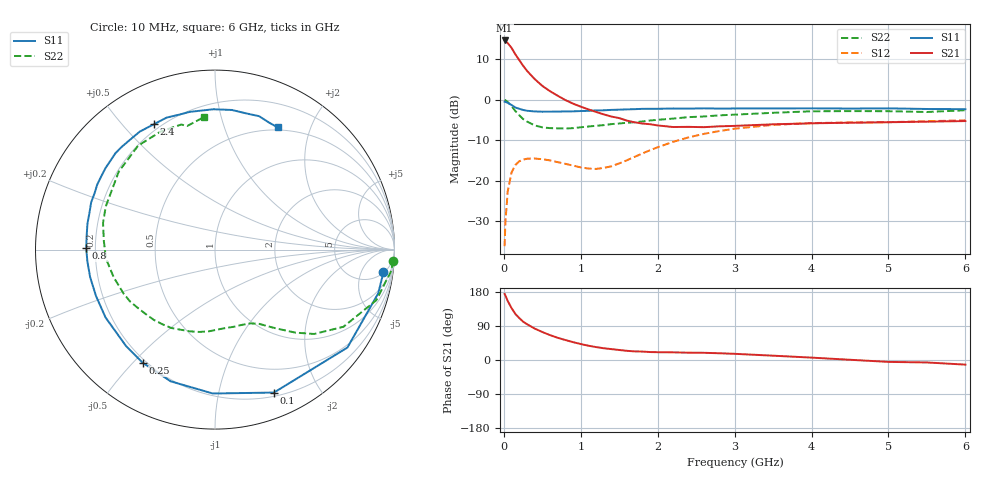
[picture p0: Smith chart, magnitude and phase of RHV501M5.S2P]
! SIEMENS Small Signal Semiconductors
! BFR106
! Si NPN RF Bipolar Junction Transistor in SOT23
! VCE = 0.5 V  IC = 1.5 mA
! Common Emitter S-Parameters:  August  1996
# GHz  S  MA  R  50
!  f  S11  S21  S12  S22
! GHz  MAG  ANG  MAG  ANG  MAG  ANG  MAG  ANG
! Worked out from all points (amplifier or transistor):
!   36 points, 10 MHz to 6 GHz, reference 50 ohm
!   highest |S21| = 14.7 dB at 10 MHz (marker M1)
!   |S21| within 3 dB of that: start of sweep to 136.2 MHz
!   unconditionally stable (mu >= 1): 770.4 MHz to end of sweep
!   at 250 MHz: K = 0.33, MSG = 11.6 dB, |S12| = -14.8 dB
!   at 1.4 GHz: K = 1.50, MAG = 2.0 dB, |S12| = -16.5 dB
!   at 6 GHz: K = 1.03, MAG = -1.1 dB, |S12| = -5.1 dB
!   S11 on the Smith chart (normalised r, x): 10 MHz: 5, -13; 100 MHz: 0.24, -1.47; 250 MHz: 0.19, -0.53; 800 MHz: 0.16, +0.01; 2.4 GHz: 0.17, +0.61; 6 GHz: 0.47, +1.53
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0.01  0.947 -7.6  5.425 174.4  0.0154 86.7  0.9962 -3.6
0.02  0.9415 -15.0  5.36 170.4  0.0302 83.4  0.9866 -7.3
0.05  0.9176 -36.5  5.041 155.9  0.0728 68.7  0.9421 -17.4
0.1  0.8616 -67.6  4.394 137.1  0.1258 52.4  0.835 -31.0
0.15  0.8018 -90.9  3.649 121.4  0.1559 39.7  0.7253 -40.4
0.2  0.7743 -108.6  3.104 110.8  0.173 31.6  0.6443 -45.9
0.25  0.7482 -122.6  2.646 101.3  0.1816 25.2  0.5779 -50.4
0.3  0.731 -132.7  2.288 94.6  0.1863 21.1  0.5379 -53.7
0.4  0.7176 -148.2  1.808 83.0  0.1873 14.8  0.4818 -59.2
0.5  0.7117 -158.6  1.487 73.9  0.1839 10.8  0.4559 -64.4
0.6  0.7124 -167.6  1.278 65.7  0.1776 8.7  0.4457 -70.0
0.8  0.7175 179.4  0.992 52.7  0.1611 8.7  0.4408 -82.2
1.1  0.7293 163.4  0.76 37.7  0.1408 18.8  0.4669 -100.7
1.6  0.7608 143.2  0.552 24.2  0.1782 44.9  0.5195 -131.2
2.2  0.7797 122.5  0.46 20.2  0.3015 46.8  0.585 -164.7
2.4  0.7771 115.8  0.462 19.3  0.3423 43.6  0.6096 -175.3
2.8  0.7779 105.0  0.469 17.8  0.4096 35.5  0.6412 166.6
3.5  0.782 90.6  0.497 11.4  0.4888 21.1  0.6901 141.0
4.5  0.7785 77.0  0.52 0.6  0.5237 4.4  0.7239 114.7
5  0.7829 71.7  0.527 -5.0  0.5284 -1.7  0.7219 105.1
5.5  0.769 66.9  0.536 -6.5  0.543 -4.5  0.7058 102.7
6  0.7653 62.9  0.545 -12.2  0.5565 -11.0  0.7421 94.6
